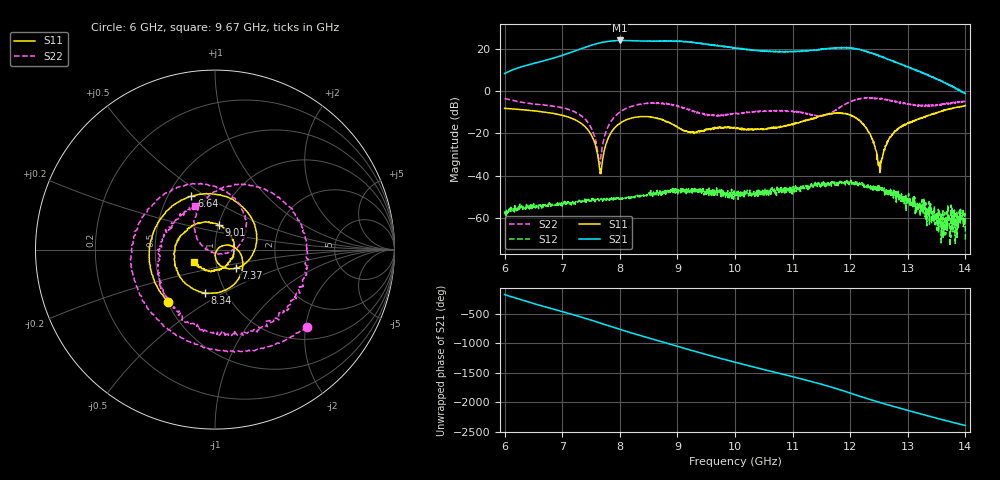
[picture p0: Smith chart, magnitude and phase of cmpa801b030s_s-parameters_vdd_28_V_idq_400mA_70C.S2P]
!Keysight Technologies,E5071C,MY46110325,B.14.03
!Date: Fri Aug 07 15:42:39 2020
!Data & Calibration Information:
!Freq	S11:SOLT2(ON)	S21:SOLT2(ON)	S12:SOLT2(ON)	S22:SOLT2(ON)
!PortZ  Port1:50+j0  Port2:50+j0
!Above PortZ is port z conversion or system Z0 setting when saving the data.
!When reading, reference impedance value at option line is always used.
# Hz S dB R 50
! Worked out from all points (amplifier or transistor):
!   1601 points, 6 GHz to 14 GHz, reference 50 ohm
!   highest |S21| = 24.0 dB at 8 GHz (marker M1)
!   |S21| within 3 dB of that: 7.424 GHz to 9.839 GHz (2.415 GHz wide, 28 % of centre)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
!   unconditionally stable (mu >= 1): start of sweep to end of sweep
!   at 7.33 GHz: K = 18.95, MAG = 20.5 dB, |S12| = -52.5 dB
!   at 10 GHz: K = 12.16, MAG = 20.9 dB, |S12| = -49.0 dB
!   at 14 GHz: K = 989.48, MAG = 1.7 dB, |S12| = -70.5 dB
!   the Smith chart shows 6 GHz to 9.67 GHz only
!   S11 on the Smith chart (normalised r, x): 6 GHz: 0.51, -0.35; 6.64 GHz: 0.65, +0.43; 7.37 GHz: 1.23, -0.26; 8.34 GHz: 0.80, -0.41; 9.01 GHz: 1.01, +0.28; 9.67 GHz: 0.79, -0.11
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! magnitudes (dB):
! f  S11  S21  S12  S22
! 6 GHz  -8.1  8.3  -57.9  -3.5
! 6.64 GHz  -9.8  14.0  -55.1  -6.4
! 7.335 GHz  -15.4  20.2  -52.3  -11.8
! 7.37 GHz  -16.2  20.4  -52.3  -12.5
! 7.535 GHz  -22.4  22.0  -51.4  -19.6
! 7.665 GHz  -38.1  22.9  -50.8  -32.4
! 7.79 GHz  -22.8  23.5  -50.8  -17.3
! 8 GHz  -15.3  24.0  -51.1  -9.9
! 8.34 GHz  -12.1  23.8  -49.3  -6.2
! 8.67 GHz  -13.0  23.7  -49.3  -5.6
! 9.01 GHz  -17.2  23.6  -49.2  -7.3
! 9.67 GHz  -17.5  21.6  -47.1  -11.5
! 10 GHz  -17.4  20.4  -49.0  -10.7
! 11.34 GHz  -13.2  19.3  -44.0  -11.3
! 12.1 GHz  -12.6  20.1  -42.9  -4.1
! 12.33 GHz  -19.7  18.4  -44.6  -3.2
! 12.52 GHz  -38.6  16.6  -47.0  -3.6
! 12.67 GHz  -22.7  15.0  -48.0  -4.1
! 12.91 GHz  -16.4  12.4  -50.7  -5.7
! 13.62 GHz  -9.2  4.2  -62.2  -6.1
! 13.93 GHz  -7.4  -0.2  -59.7  -5.2
! 14 GHz  -6.8  -1.2  -70.5  -4.6
